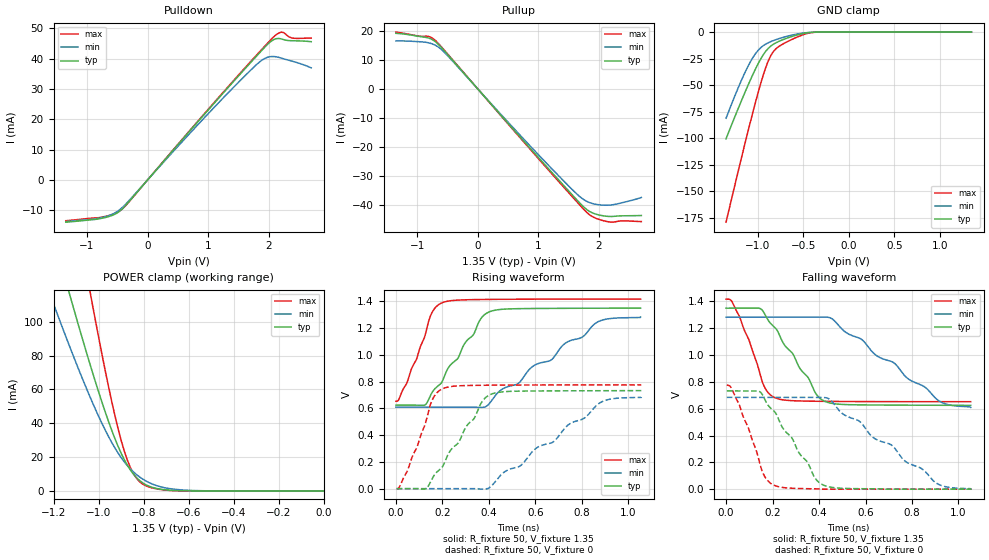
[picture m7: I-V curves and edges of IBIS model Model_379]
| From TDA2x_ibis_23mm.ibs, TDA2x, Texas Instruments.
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| Model based on original model for DDR_SEIOPB_V
|   Sub model SR111_DRV40_1P35
[model]   Model_379
|[Description]  [1.35V-I/O-X-X]
|   , ,
|[Input Load]
|[Output Drive]
|Voltage   1.35V
|Mode   I/O
Model_type   I/O
Polarity   Non-Inverting
Enable   Active-Low
Vinl =  0.585
Vinh =  0.765
Cref =  15.0000pF
Rref =  100.0000M
Vref =  0V
Vmeas =  0.675
C_comp   2p   2p   2p
[Model Spec]
Vinl   0.585   0.55125   0.61875
Vinh   0.765   0.73125   0.79875
[Receiver Thresholds]
Tslew_ac = 5n
Vth= 0.675
Vth_max= 0.709
Vth_min= 0.608
Vinh_ac= 0.175
Vinh_dc= 0.1
Vinl_ac= -0.175
Vinl_dc= -0.1
[Temperature Range]   25   125   -40
[Voltage Range]   1.35   1.2825   1.4175
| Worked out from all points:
|   slope of the pulldown table from 0 to 0.203 V, typ, clamps not added: 43 ohm
|   slope of the pullup table from 0 to 0.203 V, typ, clamps not added: 42 ohm
|   GND clamp passes 1 mA (typ) near -0.48 V on its own axis
|   POWER clamp passes 1 mA (typ) near -0.72 V on its own axis
|   rising waveform, R_fixture 50, V_fixture 1.35: 20-80 % time 164ps typ, 355ps min, 92.6ps max; typ from 0.625 V to 1.35 V
|   rising waveform, R_fixture 50, V_fixture 0: 20-80 % time 160ps typ, 346ps min, 92.6ps max; typ from 0 V to 0.733 V
|   falling waveform, R_fixture 50, V_fixture 1.35: 20-80 % time 159ps typ, 328ps min, 92.1ps max; typ from 1.35 V to 0.625 V
|   falling waveform, R_fixture 50, V_fixture 0: 20-80 % time 161ps typ, 339ps min, 92.6ps max; typ from 0.733 V to 0 V
[POWER_clamp]
-1.35V    224.4mA    165.8mA    358.5mA
-1.214V   157mA      115.5mA    250.8mA
-1.132V   117.8mA    86.59mA    187.7mA
-1.118V   111.4mA    81.92mA    177.3mA
-1.036V   74.26mA    55.16mA    116.8mA
-954.5mV  40.7mA     31.91mA    61.06mA
-900mV    22.42mA    19.79mA    30.14mA
-859.1mV  12.48mA    13.09mA    13.96mA
-804.5mV  4.85mA     7.084mA    4.132mA
-736.4mV  1.313mA    2.9mA      1.073mA
-627.3mV  101.6uA    577.3uA    45.9uA
0V        75.63nA    322.4nA    418.5nA
[Pulldown]
-1.35V    -13.93mA   -13.71mA   -13.45mA
-736.4mV  -12.58mA   -12.32mA   -12.19mA
-531.8mV  -11.22mA   -10.8mA    -10.99mA
-409.1mV  -9.378mA   -8.926mA   -9.416mA
1.145V    26.32mA    24.88mA    26.57mA
1.718V    39.05mA    36.49mA    39.37mA
1.923V    43.49mA    39.91mA    43.83mA
2.005V    45.12mA    40.54mA    45.58mA
2.086V    46.28mA    40.65mA    47.24mA
2.209V    46.44mA    40.1mA     48.7mA
2.373V    45.86mA    39.19mA    46.8mA
2.7V      45.54mA    36.91mA    46.74mA
[Pullup]
-1.35V    19.14mA    16.53mA    19.57mA
-981.8mV  18.13mA    16.28mA    18.23mA
-818.2mV  17.57mA    15.91mA    18.13mA
-736.4mV  16.82mA    15.4mA     17.33mA
-613.6mV  14.56mA    13.83mA    14.83mA
1.064V    -25.08mA   -24.06mA   -25.52mA
1.555V    -36.41mA   -34.6mA    -37.03mA
1.759V    -40.9mA    -38.29mA   -41.73mA
1.923V    -42.98mA   -39.67mA   -44.36mA
2.127V    -43.9mA    -40.1mA    -45.7mA
2.291V    -43.85mA   -39.69mA   -45.73mA
2.7V      -43.64mA   -37.43mA   -45.74mA
[GND_clamp]
-1.35V    -100.7mA   -81.27mA   -179.3mA
-1.241V   -77.31mA   -57.61mA   -140mA
-1.132V   -54.83mA   -36.31mA   -101.6mA
-1.05V    -39.08mA   -23.36mA   -74mA
-968.2mV  -25.28mA   -14.71mA   -48.34mA
-913.6mV  -18.13mA   -11.32mA   -33.52mA
-859.1mV  -13.28mA   -9.024mA   -22.35mA
-831.8mV  -11.61mA   -8.091mA   -18.64mA
-777.3mV  -9.078mA   -6.444mA   -14.07mA
-531.8mV  -1.871mA   -1.307mA   -3.441mA
-368.2mV  -88.76uA   -111.2uA   -158uA
1.35V     75.63nA    385.5nA    349.4nA
[Ramp]
dV/dt_f 0.43578696/0.15940165n 0.40496518/0.33002882n 0.45942787/92.215613p
dV/dt_r 0.44167399/0.16204354n 0.41325429/0.34889674n 0.46678551/92.873716p
R_load = 50
[Rising Waveform]
R_fixture = 50
V_fixture = 1.35
V_fixture_min = 1.2825
V_fixture_max = 1.4175
0s        624.9mV    609.4mV    653.4mV
46.84ps   624.3mV    609.3mV    789.5mV
125.3ps   626.4mV    609.3mV    1.145V
155.1ps   717.9mV    609.3mV    1.316V
198.4ps   799.1mV    609.4mV    1.389V
364.7ps   1.269V     607.2mV    1.414V
405.5ps   1.324V     644mV      1.415V
450ps     1.34V      735.3mV    1.416V
865.4ps   1.349V     1.244V     1.417V
1.053ns   1.35V      1.282V     1.417V
[Rising Waveform]
R_fixture = 50
V_fixture = 0
V_fixture_min = 0
V_fixture_max = 0
3.245ps   0V         0V         0V
49.55ps   0V         0V         132.9mV
130.7ps   0V         0V         511mV
160.2ps   88.93mV    0V         677.2mV
202.1ps   169.5mV    0V         748.1mV
371ps     651.8mV    -3.606mV   773mV
411.6ps   707.5mV    21.18mV    773.7mV
463.7ps   724.6mV    120.8mV    774.3mV
879.3ps   732.3mV    643.5mV    775.6mV
1.056ns   733mV      684.9mV    775.7mV
[Falling Waveform]
R_fixture = 50
V_fixture = 1.35
V_fixture_min = 1.2825
V_fixture_max = 1.4175
0s        1.35V      1.282V     1.417V
23.03ps   1.35V      1.283V     1.405V
57.63ps   1.35V      1.283V     1.288V
147.3ps   1.347V     1.283V     851.2mV
173.3ps   1.282V     1.283V     738.1mV
211.7ps   1.204V     1.283V     681.1mV
386.8ps   711.9mV    1.283V     655.7mV
429.6ps   652mV      1.284V     654.9mV
916.6ps   625.7mV    657.9mV    652.6mV
1.053ns   624.9mV    609.4mV    652.5mV
[Falling Waveform]
R_fixture = 50
V_fixture = 0
V_fixture_min = 0
V_fixture_max = 0
3.245ps   733mV      684.9mV    775.7mV
20.94ps   733.1mV    685mV      760mV
54.73ps   733.1mV    685mV      638.6mV
143ps     729.4mV    685mV      206.9mV
167.9ps   664.5mV    685mV      89.89mV
207.8ps   579.3mV    684.9mV    28.33mV
382.3ps   84.1mV     685.2mV    2.552mV
422.6ps   27.58mV    683.8mV    0V
906ps     0V         43.69mV    0V
1.056ns   0V         0V         0V
